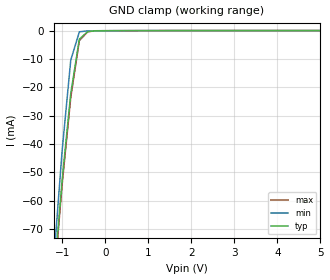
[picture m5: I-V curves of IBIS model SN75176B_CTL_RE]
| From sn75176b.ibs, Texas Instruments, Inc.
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|   Model SN75176B_CTL_RE
[Model]   SN75176B_CTL_RE
Model_type  Input
Polarity   Inverting
Vinl = 0.8
Vinh = 2.0
| variable   typ   min   max
C_comp   2.855pf   2.828pf   2.861pf
[Temperature Range]   40   0   85
| Ambient temperature   25   0   70
[Voltage Range]   5.00   4.75   5.25
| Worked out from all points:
|   GND clamp passes 1 mA (typ) near -0.45 V on its own axis
[GND Clamp]
|   Voltage   I(typ)   I(min)   I(max)
-5V       -1.045A    -1.039A    -939mA
-1.2V     -89.61mA   -82.22mA   -90.72mA
-1V       -52.86mA   -42.33mA   -54.23mA
-800mV    -22.26mA   -10.44mA   -23.61mA
-600mV    -2.986mA   -440.3uA   -3.52mA
-400mV    -325.3uA   -81.24uA   -363.4uA
-200mV    -64.28uA   -63.19uA   -69.55uA
5V        2.791nA    298.9pA    5nA
